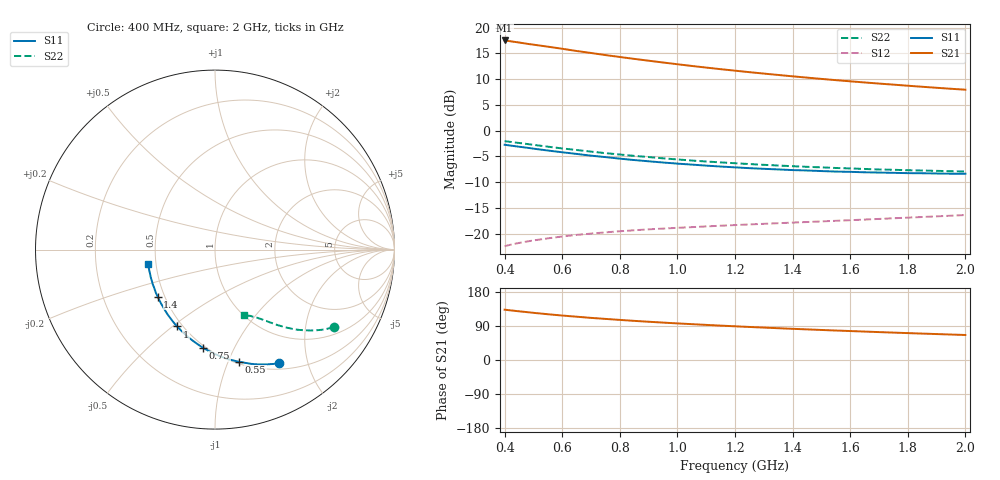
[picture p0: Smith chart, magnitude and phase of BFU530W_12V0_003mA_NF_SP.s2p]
! Filename:  P:\Prog\Test\Noise\ATS_data\Testdata_Net\06 Compressed Noise after Statistics\BFU530W_APM2013_09_A05_12p0V_003mA_NF_CM01_D.sf
! Date/Time: Tue 26/Mar/2013 18:06:02
! BFU530W_APM2013_09_A05_12p0V_1to25mA_NF_CM01_Bias3_R.sf
! Noise Parameter Data File
! BFU530W_APM2013_09_A05_12p0V_1to25mA_NF_CM01
! Date/time: Thu Mar 21 22:54:15 2013
! VAR V_out= 12.000000
! VAR I_out= 2.995000
! VAR V_in= 0.796500
! VAR I_in= 0.024200
! Device data file deembeded for feedlines and parallel
! Original file: \06 Compressed Noise after Statistics\BFU530W_APM2013_09_A05_12p0V_003mA_NF_CM01_R.sf
! Feed-files: PR019V01_070313_Feed1.s2p, PR019V01_070313_Feed2.s2p
! Parallel-file: PR019V01_070313_Par.s2p
# MHz S MA R 50
!  Freq-MHz  S11-mag  S11-arg  S21-mag  S21-arg  S12-mag  S12-arg  S22-mag  S22-arg
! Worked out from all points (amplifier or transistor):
!   37 points, 400 MHz to 2 GHz, reference 50 ohm
!   highest |S21| = 17.5 dB at 400 MHz (marker M1)
!   |S21| within 3 dB of that: start of sweep to 771.7 MHz
!   unconditionally stable (mu >= 1): nowhere
!   at 500 MHz: K = 0.36, MSG = 19.0 dB, |S12| = -21.3 dB
!   at 1.1 GHz: K = 0.70, MSG = 15.4 dB, |S12| = -18.6 dB
!   at 2 GHz: K = 0.99, MSG = 12.2 dB, |S12| = -16.4 dB
!   lowest NFmin = 0.56 dB at 400 MHz
!   S11 on the Smith chart (normalised r, x): 400 MHz: 0.58, -1.56; 550 MHz: 0.52, -1.10; 750 MHz: 0.48, -0.76; 1 GHz: 0.47, -0.52; 1.4 GHz: 0.46, -0.29; 2 GHz: 0.45, -0.08
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400  0.7279 -60.5  7.501 132.8  0.07535 58.3  0.7889 -33.2
420  0.7148 -63.0  7.372 131.0  0.0777 57.3  0.7764 -34.3
460  0.6912 -67.8  7.094 127.7  0.08193 55.5  0.7516 -36.3
500  0.6675 -72.5  6.828 124.5  0.08565 53.9  0.7266 -38.1
550  0.6398 -77.8  6.528 120.8  0.08975 52.3  0.6973 -40.3
600  0.6154 -83.1  6.229 117.3  0.09356 50.8  0.6704 -42.1
650  0.593 -87.7  5.925 114.2  0.09697 49.5  0.6474 -43.7
700  0.5704 -92.5  5.671 111.2  0.09984 48.5  0.6243 -45.3
750  0.5523 -96.8  5.41 108.5  0.1026 47.7  0.6037 -46.5
800  0.5334 -101.0  5.184 105.8  0.1052 47.0  0.5854 -47.8
850  0.5171 -105.1  4.968 103.3  0.1075 46.5  0.5675 -48.9
900  0.5029 -108.9  4.769 101.0  0.1098 46.0  0.5528 -49.9
950  0.4894 -112.6  4.582 98.7  0.1116 45.7  0.5374 -51.0
1000  0.4774 -116.2  4.406 96.6  0.1136 45.4  0.524 -51.8
1100  0.4565 -122.8  4.09 92.6  0.1172 45.3  0.5005 -53.5
1200  0.4391 -129.1  3.817 88.9  0.1207 45.3  0.4816 -55.1
1300  0.425 -135.0  3.576 85.5  0.1242 45.5  0.4647 -56.4
1400  0.4132 -140.6  3.364 82.3  0.1277 45.9  0.4506 -57.8
1500  0.4042 -145.7  3.175 79.3  0.1311 46.4  0.4389 -59.3
1600  0.3972 -150.7  3.009 76.4  0.1347 47.0  0.4288 -60.6
1750  0.3885 -157.6  2.792 72.3  0.1406 48.1  0.4159 -62.5
2000  0.381 -168.2  2.494 66.0  0.1512 49.9  0.4009 -66.1
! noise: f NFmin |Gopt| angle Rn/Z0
400  0.5594  0.3625  26.65  0.1493
460  0.5751  0.3508  31.23  0.1467
600  0.628  0.3572  39.13  0.1487
800  0.6647  0.3285  52.34  0.1352
1000  0.6976  0.3239  66.16  0.1332
1200  0.7452  0.3195  79.83  0.1242
1400  0.8077  0.3201  93.36  0.1078
1600  0.7566  0.3242  107.3  0.095
1800  0.8377  0.3387  120.6  0.0883
2000  0.8926  0.3407  136  0.0772
